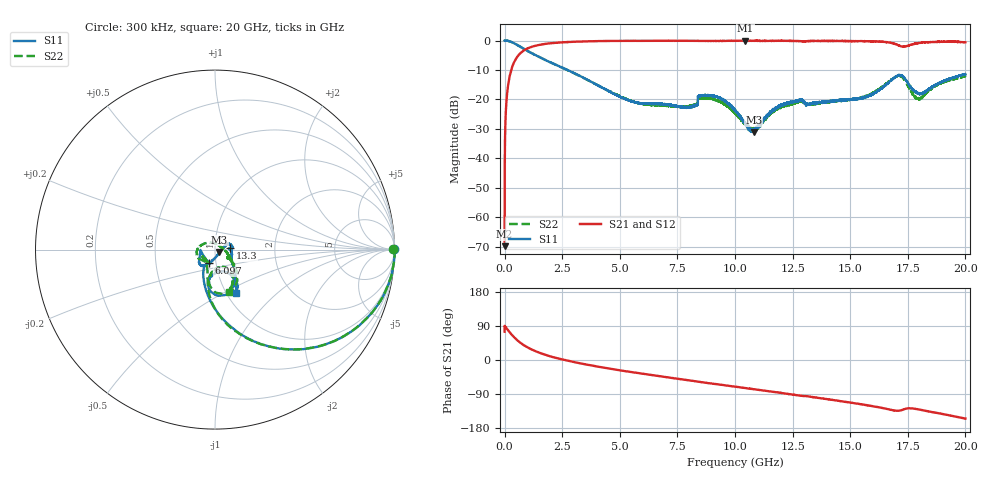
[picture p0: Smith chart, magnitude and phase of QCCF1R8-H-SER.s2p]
!QCCF1R8
!Johanson Technology Inc.
!www.johansontechnology.com
!Test Board Conditions:
!Substrate Type  RO4350B
!Substrate Thickness  10 mil
!Substrate Dk  3.66
!TL Type: GCPW
!TL Trace Width  21 mil
!TL Gap  20 mil
!Electrode orientation  Horizontal
!DUT TOPOLOGY	SERIES
!Mounting Pad LxW  16x21 mil
# MHz S  dB  R 50
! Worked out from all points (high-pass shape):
!   20001 points, 300 kHz to 20 GHz, reference 50 ohm
!   highest |S21| = -0.05 dB at 10.45 GHz (marker M1); lowest = -69.9 dB at 300 kHz (marker M2)
!   |S21| within 3 dB of the highest: 906.9 MHz to end of sweep
!   lowest |S11| = -31.2 dB at 10.81 GHz (marker M3), VSWR 1.06, Z = 52.4 - j1.4 ohm
!   |S11| at or under -10 dB: 2.729 GHz to end of sweep
!   |S22| runs from -30.7 to 0.0 dB; largest |S21 - S12| = 0.027
!   S11 on the Smith chart (normalised r, x): 300 kHz: open; 6.097 GHz: 0.92, -0.14; 13.3 GHz: 1.18, +0.02; 20 GHz: 1.11, -0.58
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0.3  -0.03 0.2  -69.87 74.6  -68.30 91.4  -0.05 0.1
101.298  -0.05 -7.6  -18.62 82.1  -18.63 82.2  -0.05 -7.7
127.298  -0.09 -9.6  -16.67 80.1  -16.70 80.2  -0.09 -9.7
253.296  -0.38 -18.6  -11.02 70.8  -11.02 71.0  -0.38 -18.8
463.293  -1.12 -32.1  -6.60 57.1  -6.58 57.3  -1.15 -32.3
1504.277  -5.64 -70.2  -1.49 19.4  -1.48 19.1  -5.59 -70.3
3334.25  -12.28 -100.8  -0.33 -9.3  -0.34 -9.3  -12.36 -98.2
6097.209  -21.43 -115.1  -0.11 -37.3  -0.11 -37.2  -21.69 -135.9
6667.2  -21.60 -111.9  -0.11 -42.3  -0.11 -42.2  -22.00 -148.4
8057.179  -22.56 -158.9  -0.11 -54.1  -0.09 -54.0  -22.19 -128.0
8898.167  -18.74 -131.0  -0.11 -61.4  -0.14 -61.2  -19.73 -171.1
10000.15  -23.52 -105.2  -0.09 -70.4  -0.11 -70.1  -24.70 141.6
10447.14  -28.32 -79.1  -0.05 -74.1  -0.09 -73.8  -28.51 103.3
10814.14  -31.22 -29.0  -0.12 -77.2  -0.11 -76.9  -29.97 56.5
11965.12  -22.28 22.8  -0.10 -86.6  -0.13 -86.6  -22.75 -17.0
13302.1  -21.64 5.1  -0.17 -97.3  -0.20 -97.5  -21.63 -28.1
13334.1  -21.45 5.2  -0.17 -97.5  -0.18 -97.5  -21.52 -28.2
15567.07  -19.39 -32.2  -0.26 -117.6  -0.17 -117.2  -19.32 -32.9
16667.05  -14.36 -53.6  -0.66 -130.1  -0.61 -130.7  -13.99 -50.9
17206.04  -11.76 -84.9  -1.98 -132.7  -2.06 -132.6  -12.20 -83.7
17970.03  -17.85 -83.0  -0.84 -130.4  -0.81 -129.6  -19.60 -76.7
20000  -11.43 -64.3  -0.61 -154.6  -0.49 -153.5  -12.06 -71.4
